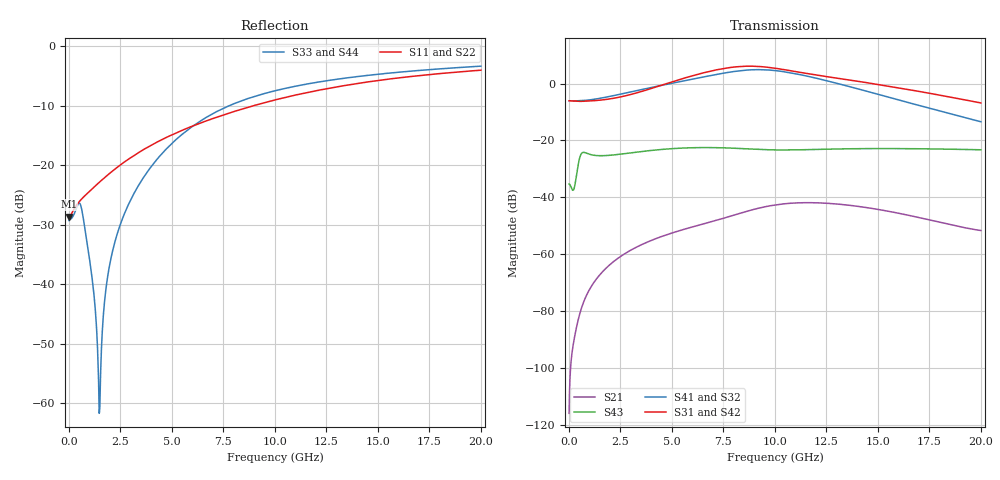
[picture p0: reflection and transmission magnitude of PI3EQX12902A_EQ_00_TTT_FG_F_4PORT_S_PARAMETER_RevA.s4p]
! NPort=4 DATA=2000 NOISE=0 GROUPDELAY=0 COMPLEX_DATAFORMAT=POLAR
! NumOfBlock=1 NumOfParam=0
! .MODEL Smodel S TSTONEFILE=PI3EQX12902A_EQ_00_TTT_FG_F_4PORT_S_PARAMETER_RevA.s4p TYPE=S
!  -- The above .MODEL line can be used for the S element in the netlist.
! The s parameter is extracted from the linear redriver, it is not bi-directional; only s(4,1)s(4,2) and s(3,1)s(3,2)
! should be the insertion loss
!Port definition:
!Port1 = input+
!Port2 = input-
!Port3 = output+
!Port4 = output-
# Hz S MA R  50
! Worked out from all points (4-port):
!   2000 points, 10 MHz to 20 GHz, reference 50 ohm
!   strongest paths, dB at 10 MHz, 5.01 GHz, 10.01 GHz, 15.01 GHz, 20 GHz:
!     S31: -6.0, 0.6, 5.4, -0.3, -6.8
!     S42: -6.0, 0.5, 5.2, -0.5, -7.0
!     S41: -6.0, 0.1, 4.6, -3.8, -13.4
!     S32: -6.0, 0.2, 4.6, -3.9, -13.6
!     S43: -35.3, -22.9, -23.3, -22.9, -23.3
!     S21: -116.0, -52.6, -42.7, -44.3, -51.7
!   lowest |S11| = -28.6 dB at 10 MHz (marker M1), VSWR 1.08, Z = 46.4 - j0.0607 ohm
!   |S11| at or under -10 dB: start of sweep to 8.96 GHz
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1e7  0.03704 -179.0  1.583e-06 51.7  0 0.0  0 0.0
     1.583e-06 51.7  0.03704 -179.0  0 0.0  0 0.0
     0.4984 -0.1  0.4985 179.9  0.03429 6.0  0.01709 -177.1
     0.4985 179.9  0.4984 -0.1  0.01709 -177.1  0.03429 6.0
1.49e9  0.0722 -133.4  0.0004287 114.9  3.744e-09 177.1  5.621e-09 -173.9
        0.0004287 114.9  0.0722 -133.4  5.622e-09 -173.8  3.745e-09 177.2
        0.5104 -0.4  0.5518 173.6  0.0008858 -60.3  0.05389 -174.9
        0.55 173.5  0.5105 -0.7  0.05389 -174.8  0.0009453 -62.8
2.6e9  0.1035 -121.8  0.0009578 104.6  2.346e-08 94.0  3.491e-08 155.0
       0.0009578 104.6  0.1035 -121.8  3.493e-08 155.1  2.342e-08 94.1
       0.5929 -0.6  0.6668 163.1  0.03555 -4.8  0.05789 178.3
       0.6634 163.2  0.5917 -1.3  0.05793 178.5  0.03548 -5.1
6.23e9  0.2206 -112.3  0.003175 73.0  1.981e-06 -28.4  1.18e-06 82.2
        0.003177 73.0  0.2206 -112.3  1.188e-06 82.4  1.976e-06 -28.3
        1.45 -41.6  1.245 99.4  0.2261 -49.0  0.07428 142.1
        1.245 99.8  1.422 -42.2  0.07469 142.2  0.2254 -49.0
8.4e9  0.2962 -112.5  0.005326 54.0  8.164e-06 -91.7  5.063e-06 26.8
       0.005344 54.0  0.2962 -112.5  5.123e-06 26.8  8.156e-06 -91.5
       2.008 -96.5  1.695 41.9  0.349 -69.5  0.07139 120.5
       1.698 42.2  1.967 -96.9  0.07183 120.4  0.3484 -69.4
1.17e10  0.4127 -116.6  0.007987 -0.9  2.15e-05 -175.9  1.496e-05 -80.3
         0.008029 -1.3  0.4127 -116.6  1.512e-05 -80.7  2.146e-05 -175.9
         1.476 -176.7  1.312 -61.3  0.486 -91.3  0.0689 101.0
         1.319 -60.9  1.439 -177.0  0.06904 100.7  0.4862 -91.2
2e10  0.6285 -131.4  0.002693 -62.8  4.726e-05 49.1  1.725e-05 115.2
      0.0026 -63.5  0.6285 -131.4  1.739e-05 114.2  4.708e-05 49.3
      0.4565 52.9  0.2086 140.9  0.6795 -119.6  0.06853 46.2
      0.2132 140.6  0.447 53.4  0.06848 46.2  0.6798 -119.6
